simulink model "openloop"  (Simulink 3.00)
settings: Solver=ode45  StartTime=0.0  StopTime=600  MaxStep=.1  RelTol=1e-3
undefined symbols (not defined in the file or in its folder): p, x0

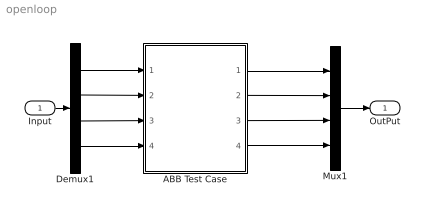
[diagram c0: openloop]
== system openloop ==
  Input : Inport  Port=1  PortWidth=-1  SampleTime=-1  DataType=auto
  ABB Test Case : Subsystem
  Demux1 : Demux  Outputs=4
  Mux1 : Mux  Inputs=4
  OutPut : Outport  Port=1
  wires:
  ABB Test Case/1(V2) -> Mux1/1
  ABB Test Case/2(V3) -> Mux1/2
  ABB Test Case/3(V4) -> Mux1/3
  ABB Test Case/4(G1Efd) -> Mux1/4
  Demux1/1 -> ABB Test Case/1(CapStep)
  Demux1/2 -> ABB Test Case/2(LoadStep)
  Demux1/3 -> ABB Test Case/3(TapVref)
  Demux1/4 -> ABB Test Case/4(faulted)
  Input/1 -> Demux1/1
  Mux1/1 -> OutPut/1

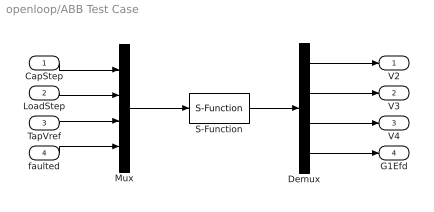
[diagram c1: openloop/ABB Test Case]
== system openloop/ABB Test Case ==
  CapStep : Inport  Port=1  PortWidth=-1  SampleTime=-1  DataType=auto
  LoadStep : Inport  Port=2  PortWidth=-1  SampleTime=-1  DataType=auto
  TapVref : Inport  Port=3  PortWidth=-1  SampleTime=-1  DataType=auto
  faulted : Inport  Port=4  PortWidth=-1  SampleTime=-1  DataType=auto
  Demux : Demux  Outputs=4
  Mux : Mux  Inputs=4
  S-Function : S-Function  FunctionName=simstr  Parameters=p,x0  PortCounts=[]  SFunctionModules=''
  V2 : Outport  Port=1
  V3 : Outport  Port=2
  V4 : Outport  Port=3
  G1Efd : Outport  Port=4
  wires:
  Mux/1 -> S-Function/1
  CapStep/1 -> Mux/1
  LoadStep/1 -> Mux/2
  TapVref/1 -> Mux/3
  faulted/1 -> Mux/4
  S-Function/1 -> Demux/1
  Demux/1 -> V2/1
  Demux/2 -> V3/1
  Demux/3 -> V4/1
  Demux/4 -> G1Efd/1
